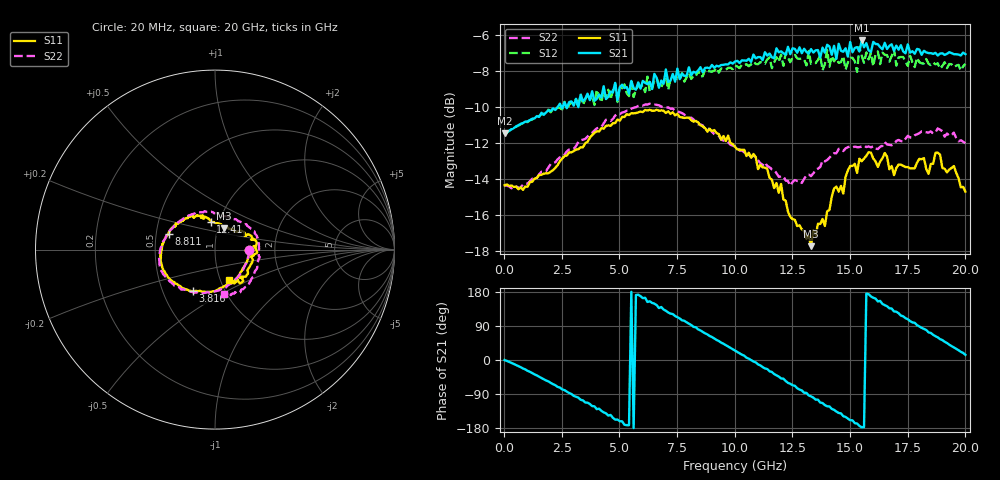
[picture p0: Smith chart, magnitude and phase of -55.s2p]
!Agilent Technologies,N5230A,US43500223,A.07.50.48
!Agilent N5230A: A.07.50.48
!Date: Thursday, October 08, 2015 19:27:09
!Correction: S11(Full 2 Port(1,2))
!S21(Full 2 Port(1,2))
!S12(Full 2 Port(1,2))
!S22(Full 2 Port(1,2))
!S2P File: Measurements: S11, S21, S12, S22:
# Hz S  RI  R 50
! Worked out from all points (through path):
!   201 points, 20 MHz to 20 GHz, reference 50 ohm
!   highest |S21| = -6.31 dB at 15.5 GHz (marker M1); lowest = -11.5 dB at 20 MHz (marker M2)
!   group delay of S21, straight-line fit = 99 ps
!   lowest |S11| = -17.7 dB at 13.31 GHz (marker M3), VSWR 1.30, Z = 53.4 + j13.1 ohm
!   |S11| at or under -10 dB: start of sweep to end of sweep
!   |S22| runs from -14.5 to -9.8 dB; largest |S21 - S12| = 0.094
!   S11 on the Smith chart (normalised r, x): 20 MHz: 1.47, -0.02; 3.816 GHz: 0.70, -0.35; 8.811 GHz: 0.59, +0.11; 12.41 GHz: 0.91, +0.29; 20 GHz: 1.09, -0.38
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2e7  0.1918 -0.00501  0.2671 -0.000977  0.2669 -0.0016  0.1919 -0.00477
1.7183e9  0.0894 -0.1863  0.1901 -0.2332  0.1912 -0.2343  0.0863 -0.1907
3.4166e9  -0.0842 -0.2296  -0.0935 -0.3147  -0.1094 -0.3013  -0.0858 -0.2418
3.8162e9  -0.1252 -0.2326  -0.1833 -0.2979  -0.182 -0.2881  -0.1266 -0.2362
5.5145e9  -0.2613 -0.1556  -0.3735 7.19e-05  -0.3775 0.00373  -0.2686 -0.1605
6.7133e9  -0.3001 -0.0729  -0.2614 0.2441  -0.255 0.2532  -0.31 -0.0782
7.7123e9  -0.2958 0.013  -0.1 0.3787  -0.0863 0.3825  -0.3041 0.00477
8.8112e9  -0.2558 0.0869  0.1546 0.376  0.1783 0.355  -0.2587 0.0978
1.001e10  -0.1908 0.1544  0.3844 0.1757  0.3845 0.1496  -0.1687 0.1783
1.13087e10  -0.0975 0.1913  0.4152 -0.1699  0.3812 -0.1692  -0.0585 0.2142
1.24076e10  -0.0232 0.1551  0.2031 -0.3936  0.1511 -0.3929  0.045 0.186
1.33067e10  0.0482 0.1208  -0.0472 -0.4553  -0.0787 -0.409  0.1278 0.1582
1.34066e10  0.0674 0.1273  -0.0721 -0.4418  -0.1089 -0.4046  0.1353 0.1568
1.4006e10  0.1271 0.1013  -0.2508 -0.398  -0.2544 -0.3772  0.1866 0.1266
1.41059e10  0.1303 0.0995  -0.2501 -0.3924  -0.2757 -0.3022  0.1933 0.1226
1.5005e10  0.2038 0.0746  -0.4468 -0.1723  -0.4004 -0.1652  0.2354 0.0701
1.55045e10  0.217 0.054  -0.4832 -0.0208  -0.4387 0.00952  0.2428 0.0383
1.67033e10  0.2105 -0.0297  -0.3389 0.322  -0.3012 0.2961  0.2401 -0.0635
1.76024e10  0.1856 -0.1062  -0.0977 0.4366  -0.0704 0.4329  0.2104 -0.1535
1.83017e10  0.1517 -0.1498  0.0834 0.4402  0.1271 0.4103  0.1703 -0.2083
1.88012e10  0.1501 -0.1825  0.2213 0.3794  0.2438 0.3397  0.1423 -0.2363
2e10  0.0756 -0.168  0.4304 0.1048  0.4114 0.0663  0.0527 -0.2452
